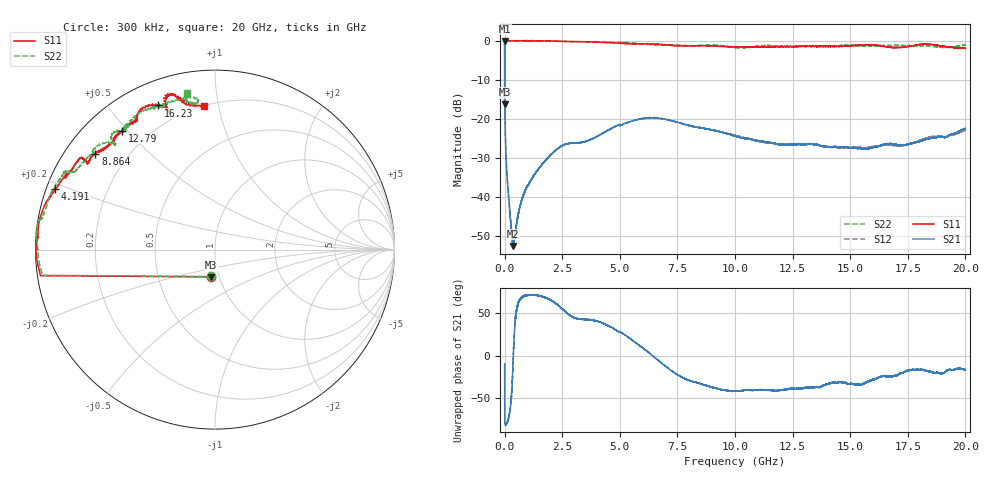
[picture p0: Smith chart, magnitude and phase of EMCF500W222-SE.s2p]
!EMCF500W222
!Johanson Technology Inc.
!www.johansontechnology.com
!Test Board Conditions:
!Substrate Type  RO4350B
!Substrate Thickness  6.6 mil
!Substrate Dk  3.66
!TL Type: GCPW
!TL Trace Width  13 mil
!TL Gap  7.5 mil
!PART MODE SINGLE ENDED (AKA BYPASS)
!DUT TOPOLOGY	SERIES-SHUNT
# MHz S  dB  R 50
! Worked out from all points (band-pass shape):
!   20001 points, 300 kHz to 20 GHz, reference 50 ohm
!   highest |S21| = -0.12 dB at 300 kHz (marker M1); lowest = -52.5 dB at 370.3 MHz (marker M2)
!   |S21| within 3 dB of the highest: start of sweep to 1.947 MHz
!   lowest |S11| = -16.3 dB at 300 kHz (marker M3), VSWR 1.36, Z = 45.7 - j14.2 ohm
!   |S11| at or under -10 dB: start of sweep to 864.4 kHz
!   |S22| runs from -16.4 to 0.0 dB; largest |S21 - S12| = 0.0038
!   S11 on the Smith chart (normalised r, x): 300 kHz: 0.91, -0.28; 4.191 GHz: 0.03, +0.18; 8.864 GHz: 0.09, +0.35; 12.79 GHz: 0.11, +0.48; 16.23 GHz: 0.11, +0.68; 20 GHz: 0.20, +0.91
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0.3  -16.27 -98.4  -0.12 -9.5  -0.10 -9.4  -16.39 -98.6
101.298  -0.04 -179.4  -34.12 -79.5  -34.08 -79.8  -0.12 -179.4
132.298  -0.03 -179.9  -36.79 -77.1  -36.72 -77.5  -0.11 -179.8
276.296  -0.04 179.2  -47.01 -54.0  -46.85 -54.7  -0.07 178.4
370.294  -0.04 178.5  -52.45 -3.3  -51.84 -7.2  -0.07 177.7
809.288  -0.07 176.5  -39.48 70.5  -39.55 70.3  0.00 174.3
1364.28  -0.09 174.9  -33.60 71.4  -33.61 71.6  -0.07 170.5
2377.264  -0.15 166.3  -27.27 58.3  -27.23 58.0  -0.19 168.8
3334.25  -0.28 162.6  -25.96 43.0  -26.01 42.9  -0.28 162.2
4191.237  -0.44 159.3  -23.87 39.2  -23.87 39.1  -0.41 156.5
6667.2  -0.96 145.4  -19.83 -5.3  -19.79 -5.5  -1.05 148.6
8864.167  -1.39 141.4  -22.66 -35.8  -22.71 -35.9  -1.15 141.0
10000.15  -1.62 137.0  -24.39 -41.6  -24.21 -41.2  -1.78 133.7
12788.11  -1.51 127.9  -26.48 -39.0  -26.32 -38.8  -1.40 126.5
13334.1  -1.48 124.1  -26.45 -37.4  -26.34 -37.6  -1.48 125.1
14436.08  -1.48 121.2  -27.22 -32.2  -27.34 -32.1  -1.36 123.5
15332.07  -1.17 119.5  -27.50 -33.9  -27.32 -32.6  -1.28 112.4
16228.06  -1.29 111.4  -26.96 -25.7  -26.95 -27.9  -1.36 110.6
16667.05  -1.68 108.9  -26.32 -24.1  -26.68 -25.6  -1.27 112.6
17367.04  -1.63 108.6  -26.64 -18.9  -26.74 -17.7  -1.32 111.1
18621.02  -1.07 104.7  -24.74 -20.0  -24.50 -20.6  -1.48 97.2
20000  -1.91 94.3  -22.41 -16.7  -22.79 -15.9  -1.08 100.2
